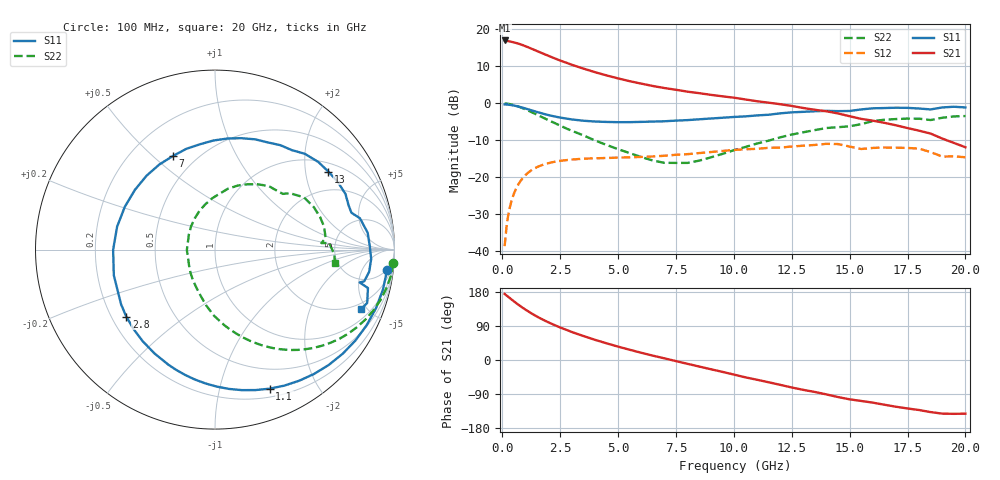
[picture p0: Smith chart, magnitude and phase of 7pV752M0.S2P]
! Infineon Technologies  Discrete & RF Semiconductors
! bfp620
! VCE = 0.75 V,  IC =  2.0 mA
! Common Emitter S-Parameters:  Sep 2002
# GHz  S  MA  R  50
!  f  S11  S21  S12  S22
! GHz  MAG  ANG  MAG  ANG  MAG  ANG  MAG  ANG
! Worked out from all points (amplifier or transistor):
!   59 points, 100 MHz to 20 GHz, reference 50 ohm
!   highest |S21| = 17.0 dB at 100 MHz (marker M1)
!   |S21| within 3 dB of that: start of sweep to 1.554 GHz
!   unconditionally stable (mu >= 1): 5.849 GHz to 15.87 GHz; 17.08 GHz to end of sweep
!   at 1 GHz: K = 0.17, MSG = 17.4 dB, |S12| = -19.4 dB
!   at 5.5 GHz: K = 0.96, MSG = 10.3 dB, |S12| = -14.6 dB
!   at 20 GHz: K = 1.73, MAG = -3.6 dB, |S12| = -14.6 dB
!   S11 on the Smith chart (normalised r, x): 100 MHz: 5, -15; 1.1 GHz: 0.28, -1.43; 2.8 GHz: 0.26, -0.32; 7 GHz: 0.37, +0.58; 13 GHz: 1.27, +2.68; 20 GHz: 1.58, -4.60
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0.1  0.9655 -6.8  7.045 174.3  0.0118 83.0  0.9969 -4.4
0.2  0.962 -13.3  6.949 169.5  0.0243 82.0  0.9899 -8.7
0.3  0.9546 -19.9  6.853 164.6  0.0367 78.6  0.9784 -12.9
0.6  0.918 -39.2  6.511 150.2  0.071 66.9  0.9244 -24.9
0.8  0.8859 -51.4  6.221 141.3  0.0905 59.6  0.8781 -32.2
1.1  0.8326 -68.5  5.725 129.1  0.1145 49.8  0.8017 -41.9
1.5  0.7636 -89.2  5.07 114.6  0.1375 38.9  0.7006 -53.0
1.9  0.705 -107.6  4.495 102.1  0.1529 30.1  0.6109 -62.1
2.4  0.6504 -128.2  3.882 88.4  0.1654 21.3  0.5168 -72.0
2.8  0.6194 -142.9  3.494 78.8  0.1715 15.4  0.4525 -79.4
3.5  0.5817 -165.7  2.943 63.3  0.1789 6.9  0.3689 -90.8
4  0.5676 -179.9  2.631 53.3  0.181 1.9  0.3158 -98.8
5  0.5562 154.5  2.167 35.3  0.1847 -5.5  0.2404 -114.7
6  0.5612 132.8  1.843 19.1  0.189 -11.4  0.1884 -136.3
7  0.5719 114.2  1.606 4.4  0.1958 -16.2  0.1573 -162.5
8.5  0.608 90.8  1.369 -17.2  0.2128 -24.3  0.1682 150.0
10.5  0.6658 63.7  1.126 -45.8  0.2395 -38.9  0.2574 102.3
13  0.7668 34.5  0.864 -78.8  0.2678 -58.0  0.4064 63.6
13.5  0.7808 28.9  0.817 -84.4  0.2742 -62.6  0.4347 56.9
15  0.7875 15.1  0.669 -103.8  0.2608 -82.7  0.489 39.4
17  0.8718 -3.4  0.505 -123.3  0.2514 -93.8  0.6129 17.2
20  0.8795 -22.1  0.255 -141.6  0.1869 -114.2  0.6725 -6.3
